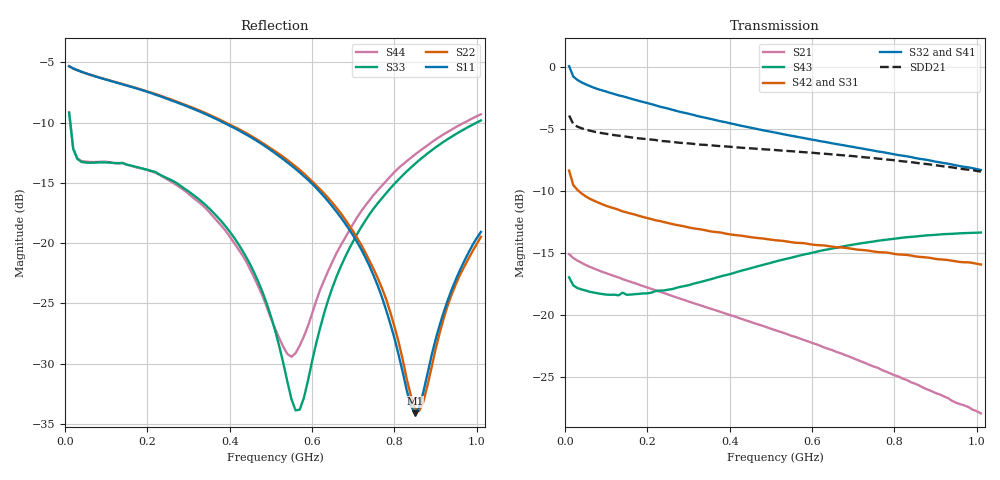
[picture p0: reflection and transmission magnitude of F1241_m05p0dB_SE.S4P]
! Integrated Device Technology
! Corporate Headquarters
! 6024 Silver Creek Valley Road
! San Jose, CA 95138  USA
! Phone:  1-408-284-8200
! Toll Free:  1-800-223-1366
! Webpage:  http://www.idt.com/
! Timing and RF Division
! 515 Groton Road, Suite 102
! Westford, MA 01886-6024
! Device:  F1241
! Description: Dual Intermediate Frequency Digital Variable Gain Amplifier
! Frequency:  10.0 -  500.00 MHz
! Package:  5x5 mm QFN Plastic Package: 32 pin
! Ports:  8 RF, 20 DC
!  Pin  1  = GA3  Pin 17  = RF OUT_B+
!  Pin  2  = GA4  Pin 18  = RF OUT_B-
!  Pin  3  = GA5  Pin 19  = STBY_B
!  Pin  4  = ISET_A  Pin 20  = Ground
!  Pin  5  = ISET_B  Pin 21  = Ground
!  Pin  6  = GB5  Pin 22  = STB_A
!  Pin  7  = GB4  Pin 23  = RF OUT_A-  = Port 4
!  Pin  8  = GB3  Pin 24  = RF OUT_A+  = Port 3
!  Pin  9  = GB2  Pin 25  = NO CONNECT
!  Pin 10  = GB1  Pin 26  = NO CONNECT
!  Pin 11  = RF IN_B+  Pin 27  = VCC
!  Pin 12  = RF IN_B-  Pin 28  = Ground
!  Pin 13  = Ground  Pin 29  = RF IN_A-  = Port 2
!  Pin 14  = VCC  Pin 30  = RF IN_A+  = Port 1
!  Pin 15  = NO CONNECT  Pin 31  = GA1
!  Pin 16  = NO CONNECT  Pin 32  = GA2
! State:  25
! Gain State:  -5.0 dB
! Voltages:  Vcc = +5.00 Volts  Icc approximately 160.0 mA or 80 mA per channel.
! Data:  The device was measured on a custom evaluation board which has
!  individual transmission lines to the RF pins.  Data was collected
!  using a calibrated network analyzer.  The evaluation board was
!  de-embedded using a port reference technique.
!  The reference plane is the edge of the package pin.
!  Only Channel A was measured.
!  This data is in single-ended operation.  If your needs are balanced
!  or differential S-parameters then this file needs to be used a
!  linear simulator.
! Misc:  Lot Code  160028MY
!  Action Tracker AT004
! Date Measured:  2014-08-14
! Date:  2014-08-28  MJV
! Note:
!  Integrated Device Technology supplies this data as a sample of measured
!  data at the package pin for this product.  Your particular data for this
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# Hz S dB R 50
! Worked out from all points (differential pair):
!   101 points, 10 MHz to 1.01 GHz, reference 50 ohm
!   strongest paths, dB at 10 MHz, 260 MHz, 510 MHz, 760 MHz, 1.01 GHz:
!     S32: 0.1, -3.4, -5.3, -6.8, -8.3
!     S41: 0.1, -3.5, -5.4, -7.0, -8.6
!     S42: -8.3, -12.6, -13.9, -14.9, -15.9
!     S31: -8.4, -12.7, -14.0, -15.0, -16.0
!     S43: -16.9, -17.9, -15.7, -14.0, -13.3
!     S21: -15.1, -18.4, -21.2, -24.2, -27.9
!   taken as a pair (ports 2,1 in; 3,4 out), SDD21 dB: -3.9, -6.0, -6.7, -7.4, -8.4
!   lowest |S11| = -34.1 dB at 850 MHz (marker M1), VSWR 1.04, Z = 51.4 + j1.42 ohm
!   |S11| at or under -10 dB: 384.8 MHz to end of sweep
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1e7  -5.33 -5.7  -15.06 -10.3  -33.96 -2.9  -24.82 6.9
     -15.07 -10.3  -5.32 -5.6  -24.84 6.6  -34.02 -2.5
     -8.35 157.0  0.07 167.2  -9.19 -42.5  -16.98 178.9
     0.12 167.3  -8.34 157.1  -16.94 178.9  -9.14 -42.3
6e7  -6.03 -8.8  -16.08 -14.1  -35.01 -7.1  -25.29 -5.9
     -16.09 -14.1  -6.03 -8.4  -25.30 -6.0  -35.11 -7.3
     -10.60 151.3  -1.53 163.2  -13.33 -9.5  -18.16 163.5
     -1.49 162.9  -10.61 151.4  -18.10 163.3  -13.27 -9.3
4e8  -10.26 -24.3  -19.95 -39.8  -36.28 0.2  -26.41 -19.6
     -19.97 -40.0  -10.16 -22.4  -26.20 -19.3  -36.20 -1.3
     -13.55 71.8  -4.52 120.2  -19.04 -15.2  -16.77 106.0
     -4.60 119.0  -13.48 71.1  -16.69 105.7  -19.45 -10.2
5.6e8  -13.85 -28.1  -21.72 -46.4  -35.29 2.5  -26.32 -26.0
       -21.74 -46.7  -13.65 -25.5  -25.99 -26.0  -35.25 0.0
       -14.25 43.8  -5.60 104.2  -33.87 47.2  -15.39 83.5
       -5.72 102.8  -14.15 42.6  -15.27 83.3  -29.12 67.1
7.4e8  -21.94 -25.3  -23.89 -51.1  -33.94 0.5  -26.33 -34.7
       -24.00 -51.4  -21.50 -22.9  -25.79 -35.3  -33.97 -2.4
       -14.94 17.6  -6.68 87.2  -17.59 128.9  -14.24 60.3
       -6.89 85.8  -14.81 15.3  -14.10 60.1  -16.42 122.8
8.5e8  -34.11 44.3  -25.42 -51.7  -33.16 -3.2  -26.43 -40.4
       -25.50 -51.5  -33.71 38.0  -25.74 -41.2  -33.12 -5.7
       -15.38 3.9  -7.33 77.2  -13.43 127.1  -13.80 47.4
       -7.57 75.9  -15.25 1.0  -13.65 47.3  -12.66 123.0
1.01e9  -19.07 122.0  -27.73 -47.4  -32.14 -9.9  -26.66 -48.4
        -27.89 -47.1  -19.48 122.9  -25.80 -49.9  -32.11 -12.6
        -16.02 -13.4  -8.29 63.3  -9.83 122.8  -13.49 30.6
        -8.58 62.3  -15.90 -17.0  -13.33 30.5  -9.32 119.0
